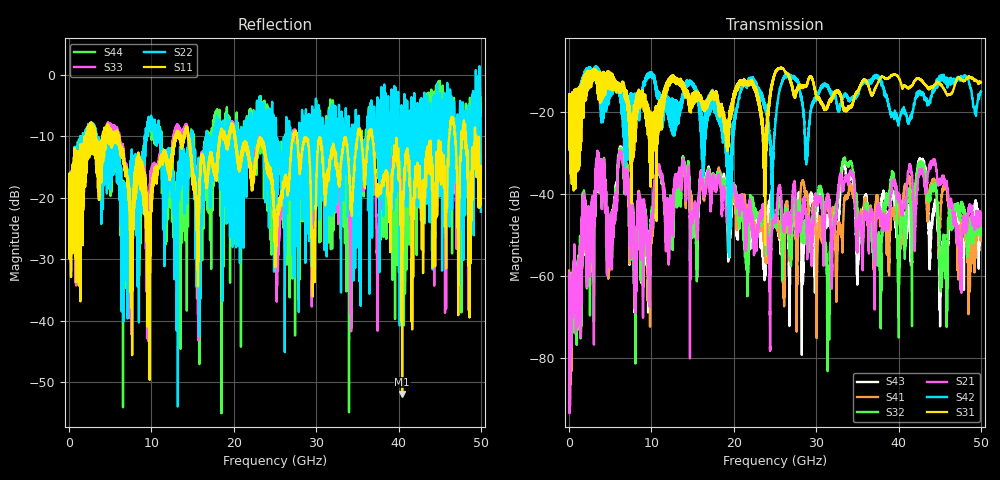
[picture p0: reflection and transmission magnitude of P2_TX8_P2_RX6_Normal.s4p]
!Keysight Technologies,N5225B,MY57041031,A.13.20.10
!Date: Friday, May 31, 2019 11:36:34
!Correction: S11(Full 4 Port(1,2,3,4))
!S12(Full 4 Port(1,2,3,4))
!S13(Full 4 Port(1,2,3,4))
!S14(Full 4 Port(1,2,3,4))
!S21(Full 4 Port(1,2,3,4))
!S22(Full 4 Port(1,2,3,4))
!S23(Full 4 Port(1,2,3,4))
!S24(Full 4 Port(1,2,3,4))
!S31(Full 4 Port(1,2,3,4))
!S32(Full 4 Port(1,2,3,4))
!S33(Full 4 Port(1,2,3,4))
!S34(Full 4 Port(1,2,3,4))
!S41(Full 4 Port(1,2,3,4))
!S42(Full 4 Port(1,2,3,4))
!S43(Full 4 Port(1,2,3,4))
!S44(Full 4 Port(1,2,3,4))
!S4P File: Measurements: <S11,S12,S13,S14>,
!<S21,S22,S23,S24>,
!<S31,S32,S33,S34>,
!<S41,S42,S43,S44>:
# Hz S  dB  R 50.0
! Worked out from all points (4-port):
!   5000 points, 10 MHz to 50 GHz, reference 50 ohm
!   strongest paths, dB at 10 MHz, 12.51 GHz, 25.01 GHz, 37.51 GHz, 50 GHz:
!     S31: -19.4, -11.7, -10.3, -12.8, -12.8
!     S42: -19.3, -16.8, -23.8, -11.2, -15.0
!     S21: -59.1, -44.1, -45.5, -43.6, -44.9
!     S32: -71.5, -44.8, -46.2, -50.3, -48.0
!     S41: -58.6, -44.1, -47.3, -40.7, -49.4
!     S43: -60.1, -45.1, -45.5, -43.5, -45.9
!   lowest |S11| = -51.9 dB at 40.44 GHz (marker M1), VSWR 1.01, Z = 49.9 - j0.243 ohm
!   |S11| at or under -10 dB: 20.17 GHz to 27.18 GHz (7.014 GHz wide, 29.6 % of centre); 27.67 GHz to 35.04 GHz (7.369 GHz wide, 23.5 % of centre); 36.79 GHz to 46.16 GHz (9.374 GHz wide, 22.6 % of centre)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
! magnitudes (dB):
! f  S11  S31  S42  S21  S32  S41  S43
! 10 MHz  -19.5  -19.4  -19.3  -59.1  -71.5  -58.6  -60.1
! 6.25 GHz  -12.9  -15.0  -17.0  -29.8  -29.5  -29.3  -29.0
! 8.03 GHz  -15.7  -17.2  -18.6  -60.9  -58.0  -56.2  -53.4
! 10.85 GHz  -15.2  -21.6  -16.6  -34.2  -34.2  -34.0  -34.4
! 31.44 GHz  -16.1  -18.1  -13.6  -40.4  -60.9  -41.4  -45.8
! 40.44 GHz  -51.9  -14.2  -19.5  -44.4  -46.7  -46.0  -44.3
! 50 GHz  -14.9  -12.8  -15.0  -44.9  -48.0  -49.4  -45.9
